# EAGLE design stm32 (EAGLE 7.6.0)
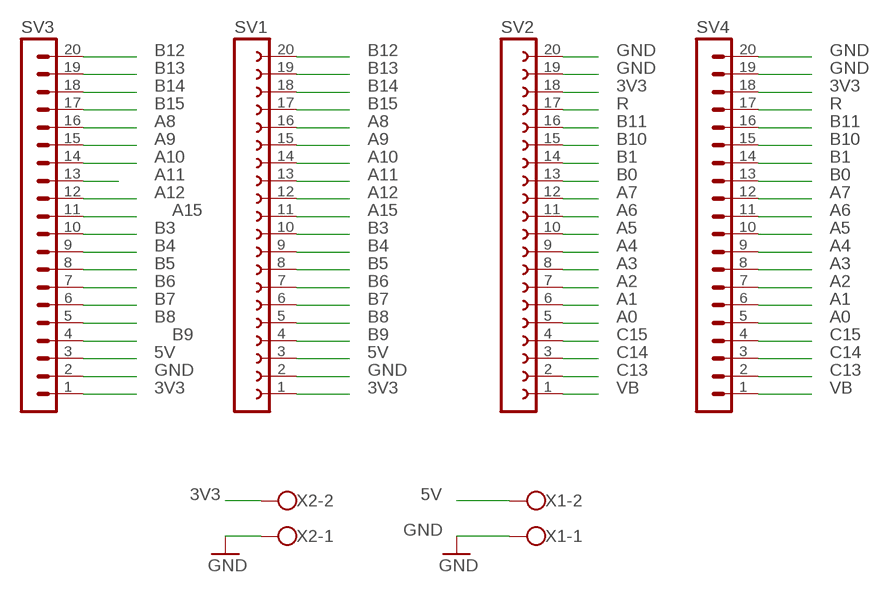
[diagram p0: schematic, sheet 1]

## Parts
SV1  FE20-1  [FE20]
SV2  FE20-1  [FE20]
SV3  MA20-1  [MA20-1]
SV4  MA20-1  [MA20-1]
X1  W237-102  [W237-102]
X2  W237-102  [W237-102]

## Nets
3V3: SV1.1 SV2.18 SV3.1 SV4.18 X2.2
5V: SV1.3 SV3.3 X1.2
A0: SV2.5 SV4.5
A1: SV2.6 SV4.6
A2: SV2.7 SV4.7
A3: SV2.8 SV4.8
A4: SV2.9 SV4.9
A5: SV2.10 SV4.10
A6: SV2.11 SV4.11
A7: SV2.12 SV4.12
A8: SV1.16 SV3.16
A9: SV1.15 SV3.15
A10: SV1.14 SV3.14
A11: SV1.13 SV3.13
A12: SV1.12 SV3.12
A15: SV1.11 SV3.11
B0: SV2.13 SV4.13
B1: SV2.14 SV4.14
B3: SV1.10 SV3.10
B4: SV1.9 SV3.9
B5: SV1.8 SV3.8
B6: SV1.7 SV3.7
B7: SV1.6 SV3.6
B8: SV1.5 SV3.5
B9: SV1.4 SV3.4
B10: SV2.15 SV4.15
B11: SV2.16 SV4.16
B12: SV1.20 SV3.20
B13: SV1.19 SV3.19
B14: SV1.18 SV3.18
B15: SV1.17 SV3.17
C13: SV2.2 SV4.2
C14: SV2.3 SV4.3
C15: SV2.4 SV4.4
GND: SV1.2 SV2.19 SV2.20 SV3.2 SV4.19 SV4.20 X1.1 X2.1
R: SV2.17 SV4.17
VB: SV2.1 SV4.1

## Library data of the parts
SV1 SV2 = con-lsta:FE20-1: FEMALE HEADER; OC_FARNELL: unknown; OC_NEWARK: unknown
SV3 SV4 = con-lstb:MA20-1: PIN HEADER; OC_FARNELL: unknown; OC_NEWARK: unknown
X1 X2 = con-wago-500:W237-102: WAGO SCREW CLAMP; MPN: 237-102; OC_FARNELL: unknown; OC_NEWARK: 70K9898

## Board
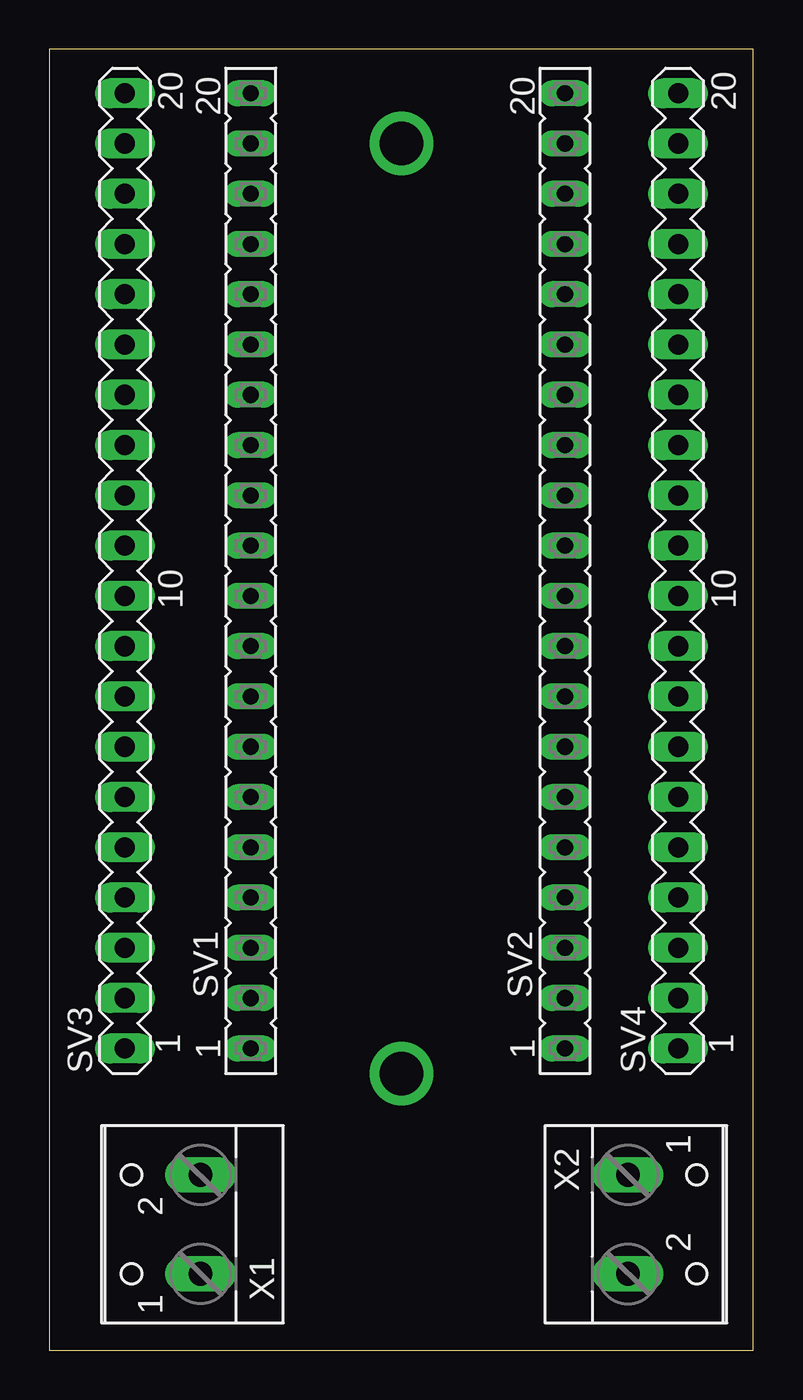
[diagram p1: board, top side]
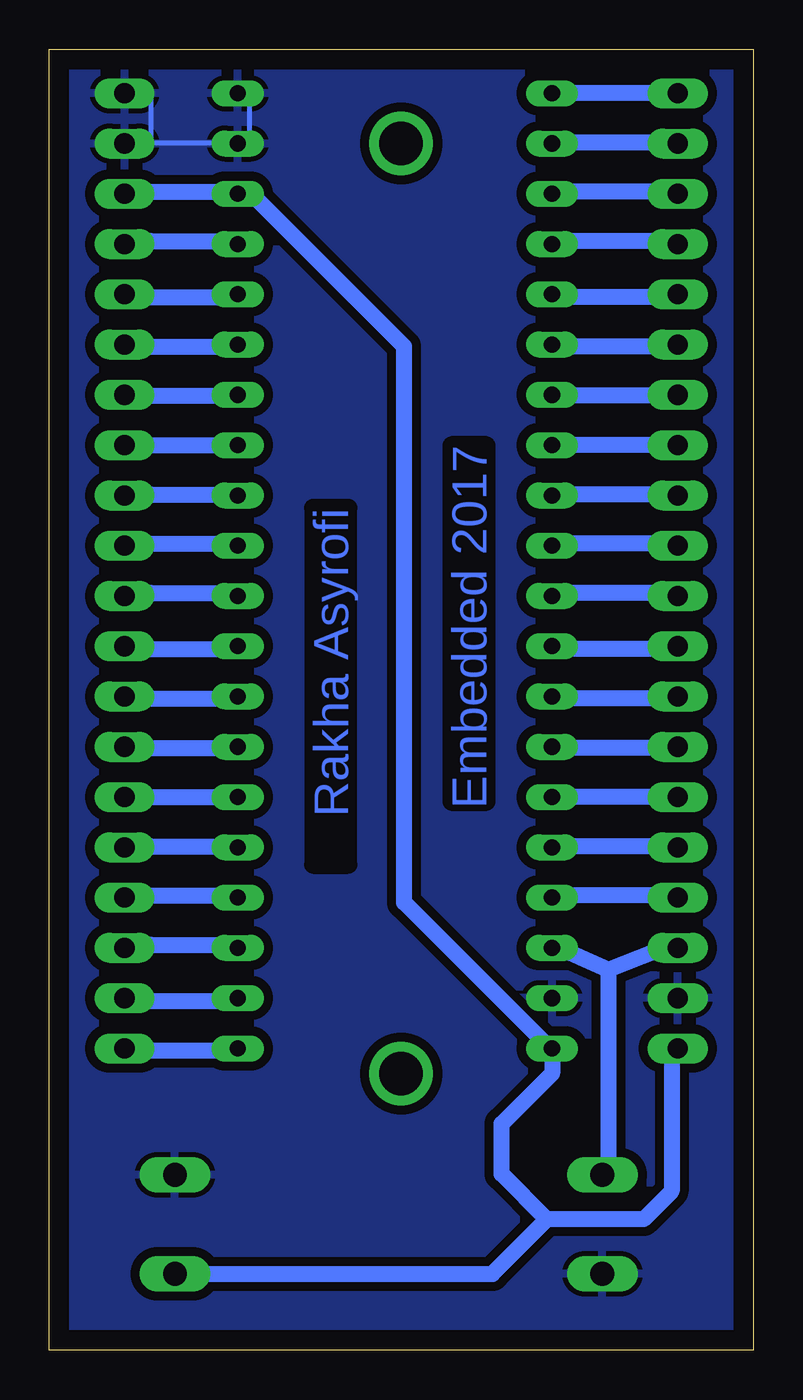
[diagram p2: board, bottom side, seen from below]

Size 35.54 x 65.71 mm. Coordinates in mm from the lower left corner, seen from the top.
Outline: 0,0 35.54,0 35.54,65.71 0,65.71 0,0
Copper layers (1*16): Top 0.035mm / dielectric 1.5mm / Bottom 0.035mm
Design rules "default *": minimum track width 10mil, minimum drill 24mil, track to track 18mil, track to pad 18mil, pad to pad 18mil, via to via 18mil, smd to smd 8mil, copper to edge 40mil, drill to drill 8mil, minimum pad ring 10mil, minimum via ring 8mil, stop-mask expansion 4mil, vias tented up to drill 0mil, thermal gap 10mil

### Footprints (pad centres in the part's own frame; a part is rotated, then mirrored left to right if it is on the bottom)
FE20 = drill 0.813 long: 1 -24.13,0; 2 -21.59,0; 3 -19.05,0; 4 -16.51,0; 5 -13.97,0; 6 -11.43,0; 7 -8.89,0; 8 -6.35,0; 9 -3.81,0; 10 -1.27,0; 11 1.27,0; 12 3.81,0; 13 6.35,0; 14 8.89,0; 15 11.43,0; 16 13.97,0; 17 16.51,0; 18 19.05,0; 19 21.59,0; 20 24.13,0
MA20-1 = drill 1.016 long: 1 -24.13,0; 2 -21.59,0; 3 -19.05,0; 4 -16.51,0; 5 -13.97,0; 6 -11.43,0; 7 -8.89,0; 8 -6.35,0; 9 -3.81,0; 10 -1.27,0; 11 1.27,0; 12 3.81,0; 13 6.35,0; 14 8.89,0; 15 11.43,0; 16 13.97,0; 17 16.51,0; 18 19.05,0; 19 21.59,0; 20 24.13,0
W237-102 = drill 1.194 long: 1 -2.5,-1.27; 2 2.5,-1.27

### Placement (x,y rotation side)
SV1  10.16,39.37 90 top
SV2  26.04,39.37 90 top
SV3  3.81,39.37 90 top
SV4  31.75,39.37 90 top
X1  6.35,6.35 90 top
X2  30.48,6.35 270 top

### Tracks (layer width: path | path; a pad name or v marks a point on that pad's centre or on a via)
3V3
  Bottom 0.254: 25.45,58.52 SV2.18 25.09,58.17 | 30.43,58.52 SV4.18 | 4.12,15.14 SV3.1 | 10.16,15.14 SV1.1
  Bottom 0.813: 30.43,58.52 25.45,58.52 | 10.41,6.6 5.54,6.6 4.12,8.03 4.12,15.14 | 25.09,58.17 17.63,50.7 17.63,22.61 10.16,15.14 10.16,13.97 12.7,11.43 12.7,8.89 10.41,6.6 | X2.2 13.17,3.85 10.41,6.6
5V
  Bottom 0.254: 10.16,20.47 SV1.3 | 4.12,20.47 SV3.3 | 7.31,9.09 X1.2
  Bottom 0.813: 4.12,20.47 7.31,19.2 | 7.31,19.2 10.16,20.47 | 7.31,19.2 7.31,9.09
A0
  Bottom 0.254: 25.45,25.45 SV2.5 | 30.43,25.45 SV4.5
  Bottom 0.813: 30.43,25.45 25.45,25.45
A1
  Bottom 0.813: SV4.6 SV2.6
A2
  Bottom 0.254: 25.45,30.43 SV2.7 | 30.43,30.43 SV4.7
  Bottom 0.813: 30.43,30.43 25.45,30.43
A3
  Bottom 0.254: 25.45,32.92 SV2.8 | 30.43,32.92 SV4.8
  Bottom 0.813: 30.43,32.92 25.45,32.92
A4
  Bottom 0.254: 25.45,35.41 SV2.9 | 30.43,35.41 SV4.9
  Bottom 0.813: 30.43,35.41 25.45,35.41
A5
  Bottom 0.254: 25.45,38.25 SV2.10 | 30.43,38.25 SV4.10
  Bottom 0.813: 30.43,38.25 25.45,38.25
A6
  Bottom 0.254: 25.45,40.74 SV2.11 | 30.43,40.74 SV4.11
  Bottom 0.813: 30.43,40.74 25.45,40.74
A7
  Bottom 0.254: 25.45,43.23 SV2.12 | 30.43,43.23 SV4.12
  Bottom 0.813: 30.43,43.23 25.45,43.23
A8
  Bottom 0.254: 10.16,53.19 SV1.16 | 4.12,53.19 SV3.16
  Bottom 0.813: 4.12,53.19 10.16,53.19
A9
  Bottom 0.254: 10.16,50.7 SV1.15 | 4.12,50.7 SV3.15
  Bottom 0.813: 4.12,50.7 10.16,50.7
A10
  Bottom 0.254: 10.16,48.21 SV1.14 | 4.12,48.21 SV3.14
  Bottom 0.813: 4.12,48.21 10.16,48.21
A11
  Bottom 0.813: SV3.13 SV1.13
A12
  Bottom 0.254: 10.16,43.23 SV1.12 | 4.12,43.23 SV3.12
  Bottom 0.813: 4.12,43.23 10.16,43.23
A15
  Bottom 0.254: 10.16,40.74 SV1.11 | 4.12,40.74 SV3.11
  Bottom 0.813: 4.12,40.74 10.16,40.74
B0
  Bottom 0.813: SV4.13 SV2.13
B1
  Bottom 0.254: 25.45,48.21 SV2.14 | 30.43,48.21 SV4.14
  Bottom 0.813: 30.43,48.21 25.45,48.21
B3
  Bottom 0.254: 10.16,38.25 SV1.10 | 4.12,38.25 SV3.10
  Bottom 0.813: 4.12,38.25 10.16,38.25
B4
  Bottom 0.254: 10.16,35.41 SV1.9 | 4.12,35.41 SV3.9
  Bottom 0.813: 4.12,35.41 10.16,35.41
B5
  Bottom 0.254: 10.16,32.92 SV1.8 | 4.12,32.92 SV3.8
  Bottom 0.813: 4.12,32.92 10.16,32.92
B6
  Bottom 0.254: 10.16,30.43 SV1.7 | 4.12,30.43 SV3.7
  Bottom 0.813: 4.12,30.43 10.16,30.43
B7
  Bottom 0.813: SV3.6 SV1.6
B8
  Bottom 0.254: 10.16,25.45 SV1.5 | 4.12,25.45 SV3.5
  Bottom 0.813: 4.12,25.45 10.16,25.45
B9
  Bottom 0.254: 10.16,22.96 SV1.4 | 4.12,22.96 SV3.4
  Bottom 0.813: 4.12,22.96 10.16,22.96
B10
  Bottom 0.254: 25.45,50.7 SV2.15 | 30.43,50.7 SV4.15
  Bottom 0.813: 30.43,50.7 25.45,50.7
B11
  Bottom 0.254: 25.45,53.19 SV2.16 | 30.43,53.19 SV4.16
  Bottom 0.813: 30.43,53.19 25.45,53.19
B12
  Bottom 0.813: SV3.20 SV1.20
B13
  Bottom 0.254: 10.16,61.01 SV1.19 | 4.12,61.01 SV3.19
  Bottom 0.813: 4.12,61.01 10.16,61.01
B14
  Bottom 0.254: 10.16,58.52 SV1.18 | 4.12,58.52 SV3.18
  Bottom 0.813: 4.12,58.52 10.16,58.52
B15
  Bottom 0.254: 10.16,56.03 SV1.17 | 4.12,56.03 SV3.17
  Bottom 0.813: 4.12,56.03 10.16,56.03
C13
  Bottom 0.254: 25.45,17.63 SV2.2 | 30.43,17.63 SV4.2
  Bottom 0.813: 30.43,17.63 25.45,17.63
C14
  Bottom 0.254: 25.45,20.47 SV2.3 | 30.43,20.47 SV4.3
  Bottom 0.813: 30.43,20.47 25.45,20.47
C15
  Bottom 0.254: 25.45,22.96 SV2.4 | 30.43,22.96 SV4.4
  Bottom 0.813: 30.43,22.96 25.45,22.96
GND
  Bottom 0.254: 25.45,61.01 25.45,63.5 SV2.20 | 30.43,61.01 30.43,63.5 SV4.20 | 30.43,61.01 25.45,61.01 | 25.45,61.01 SV2.19 | 30.43,61.01 SV4.19
  pour Bottom: 1.27,66.04 35.56,66.04 35.56,0 0,0 0,64.77
N$1  (via drill 2.2 pad 2.54)
  other vias: 17.78,60.96
N$3  (via drill 2.2 pad 2.54)
  other vias: 17.78,13.97
R
  Bottom 0.254: 25.45,56.03 SV2.17 | 30.43,56.03 SV4.17
  Bottom 0.813: 30.43,56.03 25.45,56.03
VB
  Bottom 0.254: 25.45,15.14 SV2.1 | 30.43,15.14 SV4.1
  Bottom 0.813: 30.43,15.14 25.45,15.14

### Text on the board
Bottom: Embedded 2017 | Rakha Asyrofi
